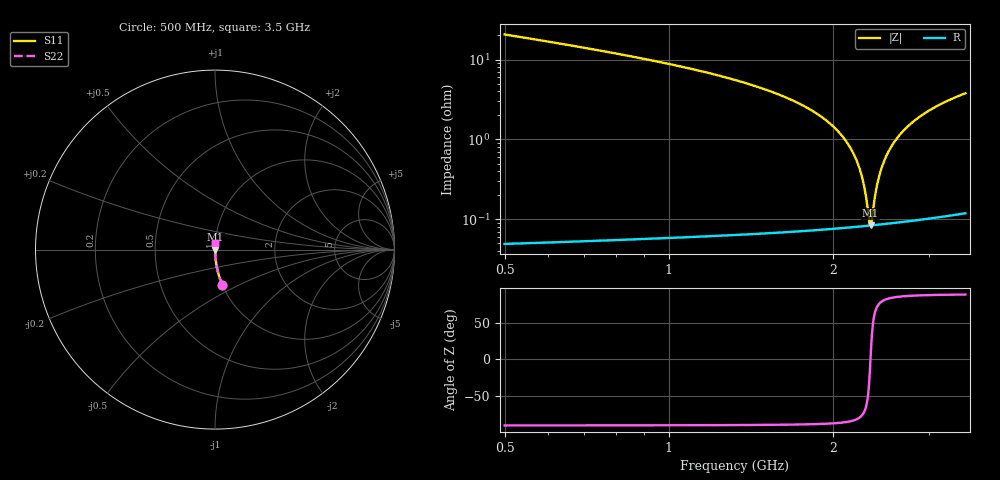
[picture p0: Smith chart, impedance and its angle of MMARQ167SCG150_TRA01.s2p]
! MMARQ167SCG150_TRA01  S-PARAMETER MODEL  ( General Type )
! Model Generated by TAIYO YUDEN Corporation (http://www.ty-top.com)
! Version 1.0
! TAIYO YUDEN Control No. 150305
! Copyright(c) 2015 TAIYO YUDEN CO.,LTD. All Rights Reserved.
! Product Description (link to TY-COMPAS)
! https://ds.yuden.co.jp/TYCOMPAS/or/detail?pn=MMARQ167SCG150JTRA01&u=M
! Products Name : Multilayer Ceramic Capacitors
! Characteristics :
!  Capacitance : 15 pF , Rated Voltage : 250V , TCC : CG / C0G
!  Case Size : 1.6 x 0.8 / 0.063 x 0.031 [mm/inch] , Thickness : 0.7 / 0.028 [mm/inch]
!  (Conditions: Temperature = 25 degC , DC Bias Current/Voltage = 0A / 0V)
! External Node Assignments :
!  1  o---| |---o  2
! GND o---------o GND
! Frequency Range : 500MHz  -  3.5GHz  [ 401 STEP ]
# MHz S RI R 50
! Freq[MHz].  S11 Real  S11 Imag  S21 Real  S21 Imag  S12 Real  S12 Imag  S22 Real  S22 Imag
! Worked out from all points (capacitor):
!   401 points, 500 MHz to 3.5 GHz, reference 50 ohm
!   read as one part in series: C = 14.8 pF near 515 MHz
!   lowest |Z| = 84 mohm at 2.345 GHz (marker M1)
!   series resonance near 2.344 GHz, so ESL is about 310 pH
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500  0.0411 -0.1973  0.9589 0.1973  0.9589 0.1973  0.0411 -0.1973
1002.5  0.00824 -0.0871  0.9918 0.0871  0.9918 0.0871  0.00824 -0.0871
1505  0.00243 -0.042  0.9976 0.042  0.9976 0.042  0.00243 -0.042
1790  0.00135 -0.0251  0.9987 0.0251  0.9987 0.0251  0.00135 -0.0251
2000  0.000976 -0.0146  0.999 0.0146  0.999 0.0146  0.000976 -0.0146
2127.5  0.000868 -0.00892  0.9991 0.00892  0.9991 0.00892  0.000868 -0.00892
2217.5  0.000835 -0.00511  0.9992 0.00511  0.9992 0.00511  0.000835 -0.00511
2270  0.00083 -0.00296  0.9992 0.00296  0.9992 0.00296  0.00083 -0.00296
2292.5  0.000831 -0.00205  0.9992 0.00205  0.9992 0.00205  0.000831 -0.00205
2330  0.000836 -0.000559  0.9992 0.000559  0.9992 0.000559  0.000836 -0.000559
2345  0.000839 2.99e-05  0.9992 -2.99e-05  0.9992 -2.99e-05  0.000839 2.99e-05
2360  0.000843 0.000616  0.9992 -0.000616  0.9992 -0.000616  0.000843 0.000616
2390  0.000853 0.00178  0.9991 -0.00178  0.9991 -0.00178  0.000853 0.00178
2420  0.000866 0.00292  0.9991 -0.00292  0.9991 -0.00292  0.000866 0.00292
2457.5  0.000886 0.00433  0.9991 -0.00433  0.9991 -0.00433  0.000886 0.00433
2502.5  0.000915 0.006  0.9991 -0.006  0.9991 -0.006  0.000915 0.006
2585  0.000982 0.00899  0.999 -0.00899  0.999 -0.00899  0.000982 0.00899
2697.5  0.0011 0.0129  0.9989 -0.0129  0.9989 -0.0129  0.0011 0.0129
2832.5  0.00128 0.0175  0.9987 -0.0175  0.9987 -0.0175  0.00128 0.0175
3005  0.00155 0.023  0.9984 -0.023  0.9984 -0.023  0.00155 0.023
3237.5  0.00201 0.0301  0.998 -0.0301  0.998 -0.0301  0.00201 0.0301
3500  0.00262 0.0377  0.9974 -0.0377  0.9974 -0.0377  0.00262 0.0377
